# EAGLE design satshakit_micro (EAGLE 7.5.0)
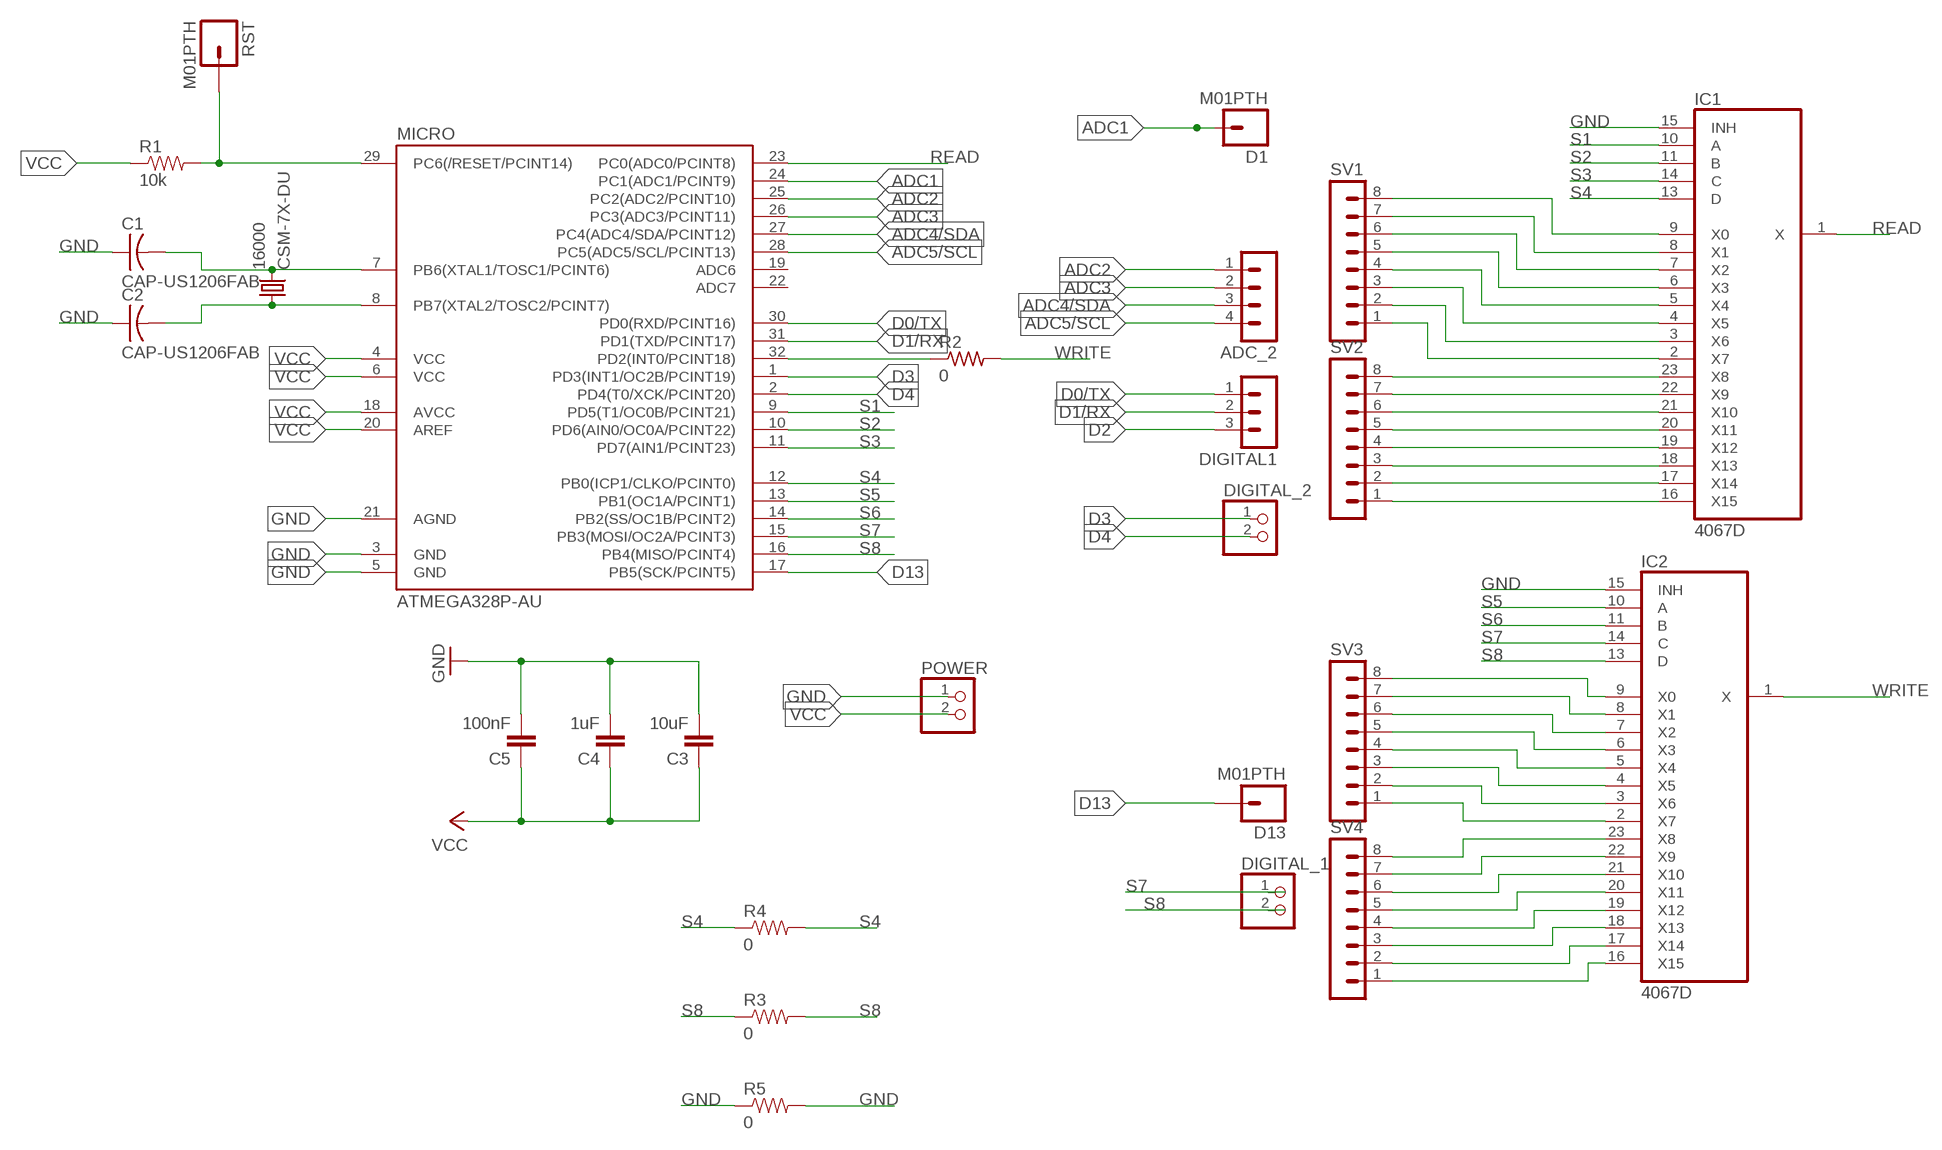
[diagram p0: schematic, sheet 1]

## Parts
16000  CSM-7X-DU  [CSM-7X-DU]
ADC_2  MA04-1  [MA04-1]
C1  CAP-US1206FAB  [C1206FAB]
C2  CAP-US1206FAB  [C1206FAB]
C3  10uF  CAP1206  [1206]
C4  1uF  CAP1206  [1206]
C5  100nF  CAP1206  [1206]
D1  M01PTH  [1X01]
D13  M01PTH  [1X01]
DIGITAL1  MA03-1  [MA03-1]
DIGITAL_1  PINHD-1X2  [1X02]
DIGITAL_2  PINHD-1X2  [1X02]
IC1  4067D  [SO24W]
IC2  4067D  [SO24W]
MICRO  ATMEGA328P-AU  ATMEGA48/88/168-AU  [TQFP32-08]
POWER  PINHD-1X2  [1X02]
R1  10k  RESISTOR1206  [1206]
R2  0  RES-US1206FAB  [R1206FAB]
R3  0  RESISTOR1206  [1206]
R4  0  RESISTOR1206  [1206]
R5  0  RESISTOR1206  [1206]
RST  M01PTH  [1X01]
SV1  MA08-1  [MA08-1]
SV2  MA08-1  [MA08-1]
SV3  MA08-1  [MA08-1]
SV4  MA08-1  [MA08-1]

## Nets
ADC1: MICRO.24(PC1(ADC1/PCINT9))
ADC2: ADC_2.1 MICRO.25(PC2(ADC2/PCINT10))
ADC3: ADC_2.2 MICRO.26(PC3(ADC3/PCINT11))
ADC4/SDA: ADC_2.3 MICRO.27(PC4(ADC4/SDA/PCINT12))
ADC5/SCL: ADC_2.4 MICRO.28(PC5(ADC5/SCL/PCINT13))
D0/TX: DIGITAL1.1 MICRO.30(PD0(RXD/PCINT16))
D1/RX: DIGITAL1.2 MICRO.31(PD1(TXD/PCINT17))
D2: DIGITAL1.3 MICRO.32(PD2(INT0/PCINT18)) R2.1
D3: DIGITAL_2.1 MICRO.1(PD3(INT1/OC2B/PCINT19))
D4: DIGITAL_2.2 MICRO.2(PD4(T0/XCK/PCINT20))
D13: D13.1 MICRO.17(PB5(SCK/PCINT5))
GND: C1.1 C2.1 C3.2 C4.2 C5.2 IC1.15(INH) IC2.15(INH) MICRO.3(GND) MICRO.5(GND) MICRO.21(AGND) POWER.1 R5.1 R5.2
N$1: 16000.1 C2.2 MICRO.8(PB7(XTAL2/TOSC2/PCINT7))
N$2: 16000.2 C1.2 MICRO.7(PB6(XTAL1/TOSC1/PCINT6))
N$3: MICRO.29(PC6(/RESET/PCINT14)) R1.2 RST.1
N$6: D1.1
N$15: IC1.9(X0) SV1.8
N$16: IC1.8(X1) SV1.7
N$17: IC1.7(X2) SV1.6
N$18: IC1.6(X3) SV1.5
N$19: IC1.5(X4) SV1.4
N$20: IC1.4(X5) SV1.3
N$21: IC1.3(X6) SV1.2
N$22: IC1.2(X7) SV1.1
N$23: IC1.23(X8) SV2.8
N$24: IC1.22(X9) SV2.7
N$25: IC1.21(X10) SV2.6
N$26: IC1.20(X11) SV2.5
N$27: IC1.19(X12) SV2.4
N$28: IC1.18(X13) SV2.3
N$31: IC1.17(X14) SV2.2
N$32: IC1.16(X15) SV2.1
N$33: IC2.9(X0) SV3.8
N$34: IC2.8(X1) SV3.7
N$35: IC2.7(X2) SV3.6
N$36: IC2.6(X3) SV3.5
N$37: IC2.5(X4) SV3.4
N$38: IC2.4(X5) SV3.3
N$39: IC2.3(X6) SV3.2
N$40: IC2.2(X7) SV3.1
N$41: IC2.23(X8) SV4.8
N$42: IC2.22(X9) SV4.7
N$43: IC2.21(X10) SV4.6
N$44: IC2.20(X11) SV4.5
N$45: IC2.19(X12) SV4.4
N$46: IC2.18(X13) SV4.3
N$47: IC2.17(X14) SV4.2
N$48: IC2.16(X15) SV4.1
READ: IC1.1(X) MICRO.23(PC0(ADC0/PCINT8))
S1: IC1.10(A) MICRO.9(PD5(T1/OC0B/PCINT21))
S2: IC1.11(B) MICRO.10(PD6(AIN0/OC0A/PCINT22))
S3: IC1.14(C) MICRO.11(PD7(AIN1/PCINT23))
S4: IC1.13(D) MICRO.12(PB0(ICP1/CLKO/PCINT0)) R4.1 R4.2
S5: IC2.10(A) MICRO.13(PB1(OC1A/PCINT1))
S6: IC2.11(B) MICRO.14(PB2(SS/OC1B/PCINT2))
S7: IC2.14(C) MICRO.15(PB3(MOSI/OC2A/PCINT3))
S8: IC2.13(D) MICRO.16(PB4(MISO/PCINT4)) R3.1 R3.2
VCC: C3.1 C4.1 C5.1 MICRO.4(VCC) MICRO.6(VCC) MICRO.18(AVCC) MICRO.20(AREF) POWER.2 R1.1
WRITE: IC2.1(X) R2.2
Unconnected: DIGITAL_1.1 DIGITAL_1.2 MICRO.19(ADC6) MICRO.22(ADC7)

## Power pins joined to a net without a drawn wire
VDD: IC1.24(VDD) IC2.24(VDD)
VSS: IC1.12(VSS) IC2.12(VSS)

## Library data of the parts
16000 = crystal:CSM-7X-DU: SMD CRYSTAL; OC_FARNELL: unknown; OC_NEWARK: unknown
ADC_2 = con-lstb:MA04-1: PIN HEADER; OC_FARNELL: unknown; OC_NEWARK: unknown
C1 C2 = fab:CAP-US
C3-C5 = 01_SparkFun:CAP: Capacitor
D1 D13 RST = 01_SparkFun:M01: Header 1
DIGITAL1 = con-lstb:MA03-1: PIN HEADER; OC_FARNELL: unknown; OC_NEWARK: unknown
DIGITAL_1 DIGITAL_2 POWER = pinhead:PINHD-1X2: PIN HEADER
IC1 IC2 = 40xx:4067: 16-channel ANALOG MULTIPLEXER
MICRO = atmega8:ATMEGA48/88/168
R1 R3-R5 = 01_SparkFun:RESISTOR: Resistor
R2 = fab:RES-US: Resistor (US Symbol)
SV1-SV4 = con-lstb:MA08-1: PIN HEADER; OC_FARNELL: unknown; OC_NEWARK: unknown

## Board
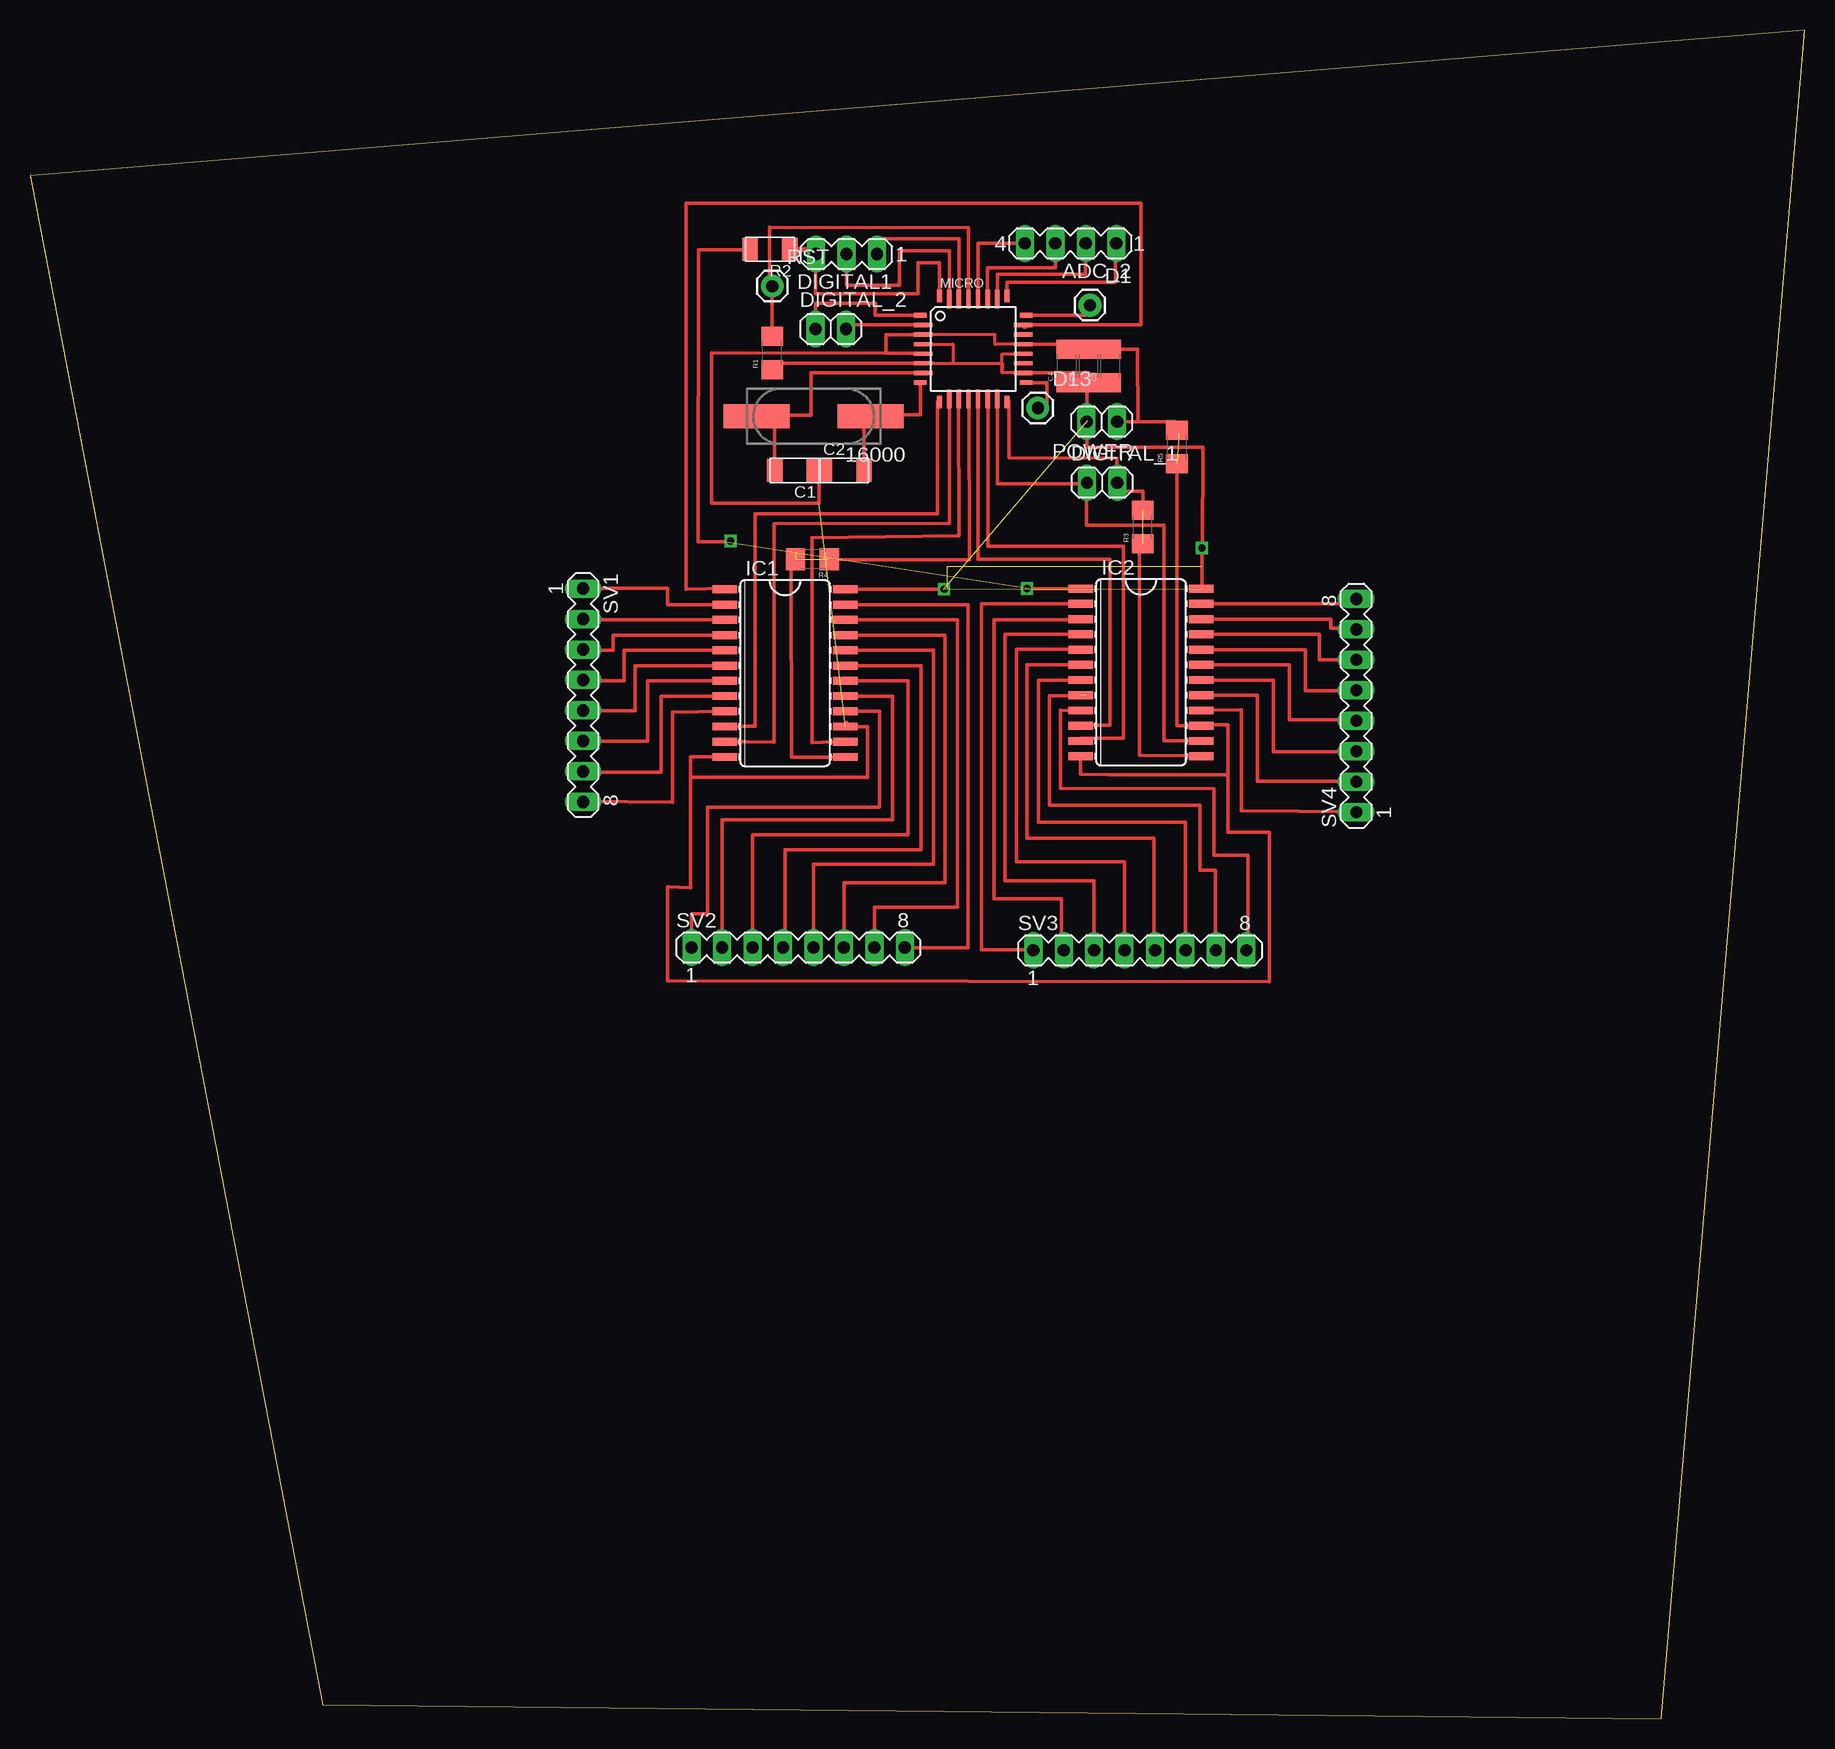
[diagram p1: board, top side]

Size 147.92 x 140.72 mm. Coordinates in mm from the lower left corner, seen from the top.
Outline: 24.38,1.17 135.98,0 147.92,140.72 0,128.56 24.38,1.17
Copper layers (1*16): Top 0.035mm / dielectric 1.5mm / Bottom 0.035mm
Design rules "default": minimum track width 10mil, minimum drill 24mil, track to track 8mil, track to pad 8mil, pad to pad 8mil, via to via 8mil, smd to smd 8mil, copper to edge 40mil, drill to drill 8mil, minimum pad ring 10mil, minimum via ring 8mil, stop-mask expansion 4mil, vias tented up to drill 0mil, thermal gap 10mil

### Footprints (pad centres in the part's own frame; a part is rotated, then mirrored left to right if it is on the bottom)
CSM-7X-DU = smd 5.5 x 2: 1 -4.75,0; 2 4.75,0
MA04-1 = drill 1.016 long: 1 -3.81,0; 2 -1.27,0; 3 1.27,0; 4 3.81,0
C1206FAB = smd 1.27 x 1.905: 1 -1.651,0; 2 1.651,0
1206 = smd 1.6 x 1.8: 1 -1.4,0; 2 1.4,0
1X01 = drill 1.016 pad 1.88: 1 0,0
MA03-1 = drill 1.016 long: 1 -2.54,0; 2 0,0; 3 2.54,0
1X02 = drill 1.016 long: 1 -1.27,0; 2 1.27,0
SO24W = smd 0.66 x 2.032: 1 -6.985,-5.029; 2 -5.715,-5.029; 3 -4.445,-5.029; 4 -3.175,-5.029; 5 -1.905,-5.029; 6 -0.635,-5.029; 7 0.635,-5.029; 8 1.905,-5.029; 9 3.175,-5.029; 10 4.445,-5.029; 11 5.715,-5.029; 12 6.985,-5.029; 13 6.985,5.029; 14 5.715,5.029; 15 4.445,5.029; 16 3.175,5.029; 17 1.905,5.029; 18 0.635,5.029; 19 -0.635,5.029; 20 -1.905,5.029; 21 -3.175,5.029; 22 -4.445,5.029; 23 -5.715,5.029; 24 -6.985,5.029
TQFP32-08 = smd 1.016 x 0.406: 1 -4.42,2.8; 8 -4.42,-2.8; 17 4.42,-2.8; 24 4.42,2.8 | smd 1.524 x 0.356: 2 -4.166,2; 3 -4.166,1.2; 4 -4.166,0.4; 5 -4.166,-0.4; 6 -4.166,-1.2; 7 -4.166,-2; 18 4.166,-2; 19 4.166,-1.2; 20 4.166,-0.4; 21 4.166,0.4; 22 4.166,1.2; 23 4.166,2 | smd 0.406 x 1.016: 9 -2.8,-4.42; 16 2.8,-4.42; 25 2.8,4.42; 32 -2.8,4.42 | smd 0.356 x 1.524: 10 -2,-4.166; 11 -1.2,-4.166; 12 -0.4,-4.166; 13 0.4,-4.166; 14 1.2,-4.166; 15 2,-4.166; 26 2,4.166; 27 1.2,4.166; 28 0.4,4.166; 29 -0.4,4.166; 30 -1.2,4.166; 31 -2,4.166
R1206FAB = smd 1.27 x 1.905: 1 -1.651,0; 2 1.651,0
MA08-1 = drill 1.016 long: 1 -8.89,0; 2 -6.35,0; 3 -3.81,0; 4 -1.27,0; 5 1.27,0; 6 3.81,0; 7 6.35,0; 8 8.89,0

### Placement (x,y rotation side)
16000  65.33,108.52 180 top
ADC_2  86.73,122.94 180 top
C1  63.73,104.02 180 top
C2  67.88,104.02 0 top
C3  90.06,112.72 90 top
C4  86.45,112.72 90 top
C5  88.25,112.72 90 top
D1  88.35,117.78 0 top
D13  84.01,109.21 0 top
DIGITAL1  68.06,122.05 180 top
DIGITAL_1  89.36,102.99 0 top
DIGITAL_2  66.74,115.8 0 top
IC1  62.93,87.12 270 top
IC2  92.61,87.19 270 top
MICRO  78.63,114.14 0 top
POWER  89.35,108.08 180 top
R1  61.86,113.81 90 top
R2  61.68,122.45 180 top
R3  92.75,99.3 90 top
R4  65.22,96.61 180 top
R5  95.6,105.97 90 top
RST  61.88,119.37 0 top
SV1  46.1,85.28 270 top
SV2  64.03,64.26 0 top
SV3  92.52,64.03 0 top
SV4  110.55,84.42 90 top

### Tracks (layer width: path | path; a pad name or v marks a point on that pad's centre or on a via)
ADC1
  Top 0.305: MICRO.24 88.08,116.94
ADC2
  Top 0.305: MICRO.25 81.43,119.69 90.49,119.69 90.49,122.89 ADC_2.1
ADC3
  Top 0.305: MICRO.26 80.63,120.35 87.98,120.35 87.98,122.91 ADC_2.2
ADC4/SDA
  Top 0.305: MICRO.27 79.83,120.91 85.46,120.91 ADC_2.3
ADC5/SCL
  Top 0.305: MICRO.28 79.03,122.96 82.9,122.96 ADC_2.4
D0/TX
  Top 0.305: MICRO.30 77.43,123.32 70.6,123.32 DIGITAL1.1
D1/RX
  Top 0.305: MICRO.31 76.63,122.3 72.49,122.3 72.49,119.46 68.06,119.46 DIGITAL1.2
D2
  Top 0.305: MICRO.32 75.83,121.31 74.03,121.31 74.03,118.72 65.5,118.72 65.5,122.02 DIGITAL1.3
  Top 0.406: R2.1 65.5,122.45 DIGITAL1.3
D3
  Top 0.305: MICRO.1 70.46,116.94 70.46,117.94 65.47,117.96 DIGITAL_2.1
D4
  Top 0.305: MICRO.2 68.35,116.14 DIGITAL_2.2
D13
  Top 0.305: MICRO.17 84.78,111.34 84.78,109.2 84.01,109.2 D13.1
GND  (2 unrouted)
  Top 0.254: MICRO.21 82.78,114.53 80.45,114.52 80.45,115.32 MICRO.3
  Top 0.279: 56.8,113.82 71.35,113.79 | 71.35,113.79 74.46,113.79 MICRO.5 | MICRO.3 71.35,115.34 71.35,113.79
  Top 0.305: MICRO.21 86.03,114.54 C4.2 C5.2 C3.2 92.32,114.12 92.35,108.09 | 92.35,108.09 POWER.1 | 56.8,113.82 56.8,101.3 65.78,101.3 65.78,103.95 66.46,103.95 66.46,104.02 C2.1 C1.1 | 92.35,108.09 95.46,108.07 95.46,107.37 R5.2 95.75,107.37 95.75,107.12 | IC2.15 95.6,82.74 R5.1
N$1
  Top 0.305: 74.16,111.21 74.21,111.21 74.21,108.66 70.08,108.66 16000.1 69.53,108.52 C2.2
  Top 0.406: MICRO.8 74.16,111.34 74.16,111.21
N$2
  Top 0.305: 16000.2 62.08,108.52 | 62.08,108.52 C1.2 | MICRO.7 65.09,112.14 65.09,108.6 62.08,108.6 62.08,108.52
N$3
  Top 0.305: 61.84,115.21 R1.2 61.86,119.35 RST.1 61.64,119.4 61.64,124.28 78.23,124.26 MICRO.29
N$7  (via drill 0.6)
  other vias: 83.11,94.18
N$8  (via drill 0.6)
  other vias: 58.4,98.13
N$9  (via drill 0.6)
  other vias: 76.21,94.11
N$10  (via drill 0.6)
  other vias: 97.7,97.55
N$15
  Top 0.305: IC1.9 53.57,83.88 53.57,76.38 46.1,76.45 SV1.8
N$16
  Top 0.305: IC1.8 52.59,85.22 52.59,78.87 46.1,78.87 SV1.7
N$17
  Top 0.305: IC1.7 51.5,86.49 51.5,81.44 46.1,81.44 SV1.6
N$18
  Top 0.305: IC1.6 50.43,87.76 50.43,84.01 SV1.5
N$19
  Top 0.305: IC1.5 49.5,89.03 49.5,86.48 46.1,86.48 SV1.4
N$20
  Top 0.305: IC1.4 48.6,90.3 48.6,89.05 46.1,89.05 SV1.3
N$21
  Top 0.305: IC1.3 46.1,91.57 SV1.2
N$22
  Top 0.305: IC1.2 53.16,92.84 53.16,94.18 46.1,94.18 SV1.1
N$23
  Top 0.305: IC1.23 78.2,92.84 78.2,64.23 72.92,64.23 SV2.8
N$24
  Top 0.305: IC1.22 77.29,91.57 77.29,67.6 70.38,67.6 SV2.7
N$25
  Top 0.305: IC1.21 76.29,90.29 76.28,69.65 67.84,69.65 SV2.6
N$26
  Top 0.305: IC1.20 75.31,89.03 75.31,71.19 65.3,71.19 SV2.5
N$27
  Top 0.305: SV2.4 62.95,64.26 62.95,72.42 74.29,72.42 74.29,87.74 69.54,87.74 IC1.19
N$28
  Top 0.305: IC1.18 73.17,86.49 73.17,73.68 60.22,73.68 SV2.3
N$31
  Top 0.305: IC1.17 71.92,85.22 71.92,74.89 57.68,74.89 SV2.2
N$32
  Top 0.305: IC1.16 70.79,83.95 70.79,75.93 56.48,75.93 56.48,67.08 55.14,67.08 SV2.1
N$33
  Top 0.305: SV3.8 101.52,64.03 101.52,71.93 98.68,71.93 98.68,77.49 85.89,77.54 85.88,84.02 87.58,84 IC2.9
N$34  (1 unrouted)
  Top 0.305: SV3.7 98.83,64.03 98.83,70.71 97.52,70.71 97.52,76.1 84.98,76.1 84.98,85.24 88.11,85.24 88.11,85.3
N$35
  Top 0.305: IC2.7 84.06,86.55 84.06,74.68 96.33,74.68 SV3.6
N$36
  Top 0.305: SV3.5 93.7,64.03 93.7,73.38 83.1,73.38 83.1,87.84 87.58,87.84 IC2.6
N$37
  Top 0.305: SV3.4 91.24,71.42 82.22,71.42 82.22,89.12 87.58,89.12 IC2.5
N$38
  Top 0.305: IC2.4 81.29,90.36 81.29,69.82 88.71,69.82 SV3.3
N$39
  Top 0.305: SV3.2 86,64.03 86,68.33 80.34,68.32 80.35,91.57 87.58,91.58 IC2.3
N$40
  Top 0.305: IC2.2 79.32,92.9 79.32,64.06 83.63,64.06 SV3.1
N$41
  Top 0.305: IC2.23 110.55,92.9 SV4.8
N$42
  Top 0.305: IC2.22 108.45,91.63 108.45,90.86 110.55,90.86 SV4.7
N$43
  Top 0.305: IC2.21 107.5,90.36 107.5,88.24 SV4.6
N$44
  Top 0.305: IC2.20 106.31,89.09 106.31,85.67 110.55,85.67 SV4.5
N$45
  Top 0.305: IC2.19 104.98,87.82 104.98,83.25 110.55,83.25 SV4.4
N$46
  Top 0.305: IC2.18 103.66,86.55 103.66,80.58 110.55,80.58 SV4.3
N$47
  Top 0.305: IC2.17 102.33,85.28 102.33,78.11 111.21,78.11 111.21,77.78 110.55,77.78 SV4.2
N$48
  Top 0.305: IC2.16 101,84.06 101,75.64 110.55,75.59 SV4.1
READ
  Top 0.305: MICRO.23 82.86,116.14 82.86,115.95 82.99,115.95 82.99,116.14 92.62,116.14 92.62,126.26 54.7,126.26 54.7,94.11 58.13,94.18 IC1.1
S1
  Top 0.305: MICRO.9 75.64,109.72 75.64,100.4 60.43,100.4 60.43,82.69 59.48,82.69 IC1.10
S2
  Top 0.305: IC1.11 59.67,81.41 59.65,81.4 62.02,81.37 62.02,99.59 76.65,99.6 MICRO.10
S3
  Top 0.305: MICRO.11 77.41,109.97 77.42,98.57 65.18,98.39 65.17,81.34 66.07,81.37 IC1.14
S4  (2 unrouted)
  Top 0.305: MICRO.12 78.29,109.94 78.31,96.59 68.5,96.59 R4.1 | IC1.13 67.96,80.1 63.48,80.1 63.44,96.17 63.83,95.97 63.83,97.18
S5
  Top 0.305: MICRO.13 79.03,96.6 90.04,96.6 90.04,82.8 87.58,82.8 IC2.10
S6
  Top 0.305: MICRO.14 79.87,109.97 79.87,97.69 91.14,97.69 91.14,81.7 87.58,81.7 IC2.11
S7
  Top 0.305: MICRO.15 80.67,109.97 | IC2.14 97.6,81.49 94.52,81.5 94.52,99.45 88.06,99.45 88.06,102.89 80.67,102.89 80.67,109.97 | 80.68,109.97 80.67,109.97
S8  (1 unrouted)
  Top 0.305: MICRO.16 81.61,109.72 81.61,105.07 90.59,105.05 90.59,102.26 92.79,102.26 R3.2 | IC2.13 97.64,80.23 92.49,80.27 92.49,97.84 R3.1
VCC
  Top 0.254: 82.18,113.76 82.18,113.74 MICRO.20 81.04,113.74 81.04,112.14 MICRO.18 | MICRO.6 | 75.15,112.95 76.93,112.95 | 76.93,112.95 81.04,112.95 81.04,112.14 MICRO.18 | MICRO.4 76.93,114.54 76.93,112.95
  Top 0.279: 84.95,112.15 88.25,112.15 C5.1
  Top 0.305: MICRO.18 | MICRO.20 82.18,113.76 | 82.79,112.11 MICRO.18 | 75.15,112.95 MICRO.6 | MICRO.6 61.86,112.95 R1.1 | 85.79,111.31 87.04,111.31 87.06,111.28 86.49,111.28 C4.1 C5.1 | POWER.2 88.11,111.18 C5.1 | C5.1 C3.1 | 84.95,112.15 MICRO.18
VDD  (4 unrouted)
  Top 0.305: IC1.24 76.15,94.11 76.15,94.06 76.14,94.06 | IC2.24 97.69,94.17 97.69,97.44 97.74,97.55 97.77,105.94 88.12,105.94 88.12,108.02 88.15,108.02 88.15,108.17 | 76.14,94.06 76.14,94.03 | 76.14,94.06 76.14,94.13
VSS
  Top 0.305: IC2.12 87.58,78.68 89.91,78.67 99.86,78.67 | 99.86,78.67 99.86,82.81 97.58,82.81 97.58,82.76 | 68.05,83.01 68.05,82.67 69.81,82.67 69.81,78.45 55.05,78.45 | 55.05,78.45 55.05,69.25 53.15,69.32 53.15,61.49 103.32,61.42 103.32,73.88 99.86,73.88 99.86,78.67 | IC1.12 55.05,80.14 55.05,78.45
WRITE  (1 unrouted)
  Top 0.305: R2.2 60.4,122.43 57.42,122.42 55.72,122.42 55.7,98.07 58.41,98.09 57.98,98.08 | IC2.1 83.26,94.17 83.26,94.18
